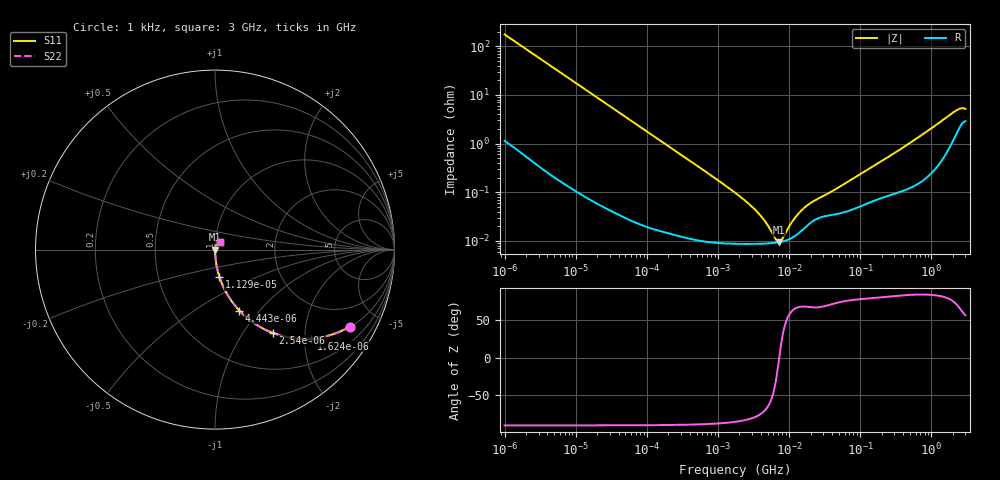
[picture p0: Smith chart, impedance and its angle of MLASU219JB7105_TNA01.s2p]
! MLASU219JB7105_TNA01  S-PARAMETER MODEL  ( Standard Model )
! Model Generated by TAIYO YUDEN Corporation (http://www.ty-top.com)
! Version 1.0
! TAIYO YUDEN Control No. 220601
! Copyright(c) 2011 TAIYO YUDEN CO.,LTD. All Rights Reserved.
! Product Description (link to TY-COMPAS)
! https://ds.yuden.co.jp/TYCOMPAS/or/detail?pn=MLASU219JB7105KTNA01&u=M
! Products Name : Multilayer Ceramic Capacitors
! Characteristics :
!  Capacitance : 1 [uF] , Rated Voltage : 50 [V] , TCC : X7R
!  Case Size : 2.0 x 1.25 / 0.079 x 0.049 [mm/inch] , Thickness : 0.85 / 0.033 [mm/inch]
!  (Conditions: Temperature = 25 [degC] , DC Bias Voltage = 0 [V])
! External Node Assignments :
!  1  o---| |---o  2
! GND o---------o GND
! Frequency Range : 1kHz  -  3GHz  [ 401 STEP ]
# MHZ S RI R 50
! Freq[MHz].  S11 Real  S11 Imag  S21 Real  S21 Imag  S12 Real  S12 Imag  S22 Real  S22 Imag
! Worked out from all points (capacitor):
!   401 points, 1 kHz to 3 GHz, reference 50 ohm
!   read as one part in series: C = 914 nF near 1.077 kHz
!   lowest |Z| = 9.4 mohm at 7.143 MHz (marker M1)
!   series resonance near 7.246 MHz, so ESL is about 530 pH
!   S11 on the Smith chart (normalised r, x): 1 kHz: 1.02, -3.48; 1.624 kHz: 1.01, -2.15; 2.54 kHz: 1.01, -1.37; 4.443 kHz: 1.00, -0.79; 11.29 kHz: 1.00, -0.31; 3 GHz: 1.06, +0.09
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0.001  0.75 -0.4298  0.25 0.4298  0.25 0.4298  0.75 -0.4298
0.001624  0.5351 -0.4956  0.4649 0.4956  0.4649 0.4956  0.5351 -0.4956
0.00254  0.3219 -0.4642  0.6781 0.4642  0.6781 0.4642  0.3219 -0.4642
0.004443  0.1356 -0.3395  0.8644 0.3395  0.8644 0.3395  0.1356 -0.3395
0.011286  0.0245 -0.1515  0.9755 0.1515  0.9755 0.1515  0.0245 -0.1515
0.01216  0.0212 -0.1411  0.9788 0.1411  0.9788 0.1411  0.0212 -0.1411
0.033275  0.00318 -0.0527  0.9968 0.0527  0.9968 0.0527  0.00318 -0.0527
0.147855  0.000305 -0.012  0.9997 0.012  0.9997 0.012  0.000305 -0.012
1.732051  8.8e-05 -0.000973  0.9999 0.000973  0.9999 0.000973  8.8e-05 -0.000973
3.651041  8.7e-05 -0.000367  0.9999 0.000367  0.9999 0.000367  8.7e-05 -0.000367
4.739869  8.82e-05 -0.000217  0.9999 0.000217  0.9999 0.000217  8.82e-05 -0.000217
6.387174  9.15e-05 -6.32e-05  0.9999 6.32e-05  0.9999 6.32e-05  9.15e-05 -6.32e-05
7.143107  9.38e-05 -7.1e-06  0.9999 7.1e-06  0.9999 7.1e-06  9.38e-05 -7.1e-06
7.988506  9.7e-05 4.92e-05  0.9999 -4.92e-05  0.9999 -4.92e-05  9.7e-05 4.92e-05
10.76485  0.000114 0.000206  0.9999 -0.000206  0.9999 -0.000206  0.000114 0.000206
13.46371  0.000142 0.000332  0.9999 -0.000332  0.9999 -0.000332  0.000142 0.000332
21.06097  0.000249 0.000578  0.9998 -0.000578  0.9998 -0.000578  0.000249 0.000578
44.39505  0.000352 0.00108  0.9996 -0.00108  0.9996 -0.00108  0.000352 0.00108
256.0921  0.000888 0.00539  0.9991 -0.00539  0.9991 -0.00539  0.000888 0.00539
2144.796  0.0155 0.0427  0.9845 -0.0427  0.9845 -0.0427  0.0155 0.0427
2584.342  0.025 0.045  0.975 -0.045  0.975 -0.045  0.025 0.045
3000  0.0297 0.0404  0.9703 -0.0404  0.9703 -0.0404  0.0297 0.0404
